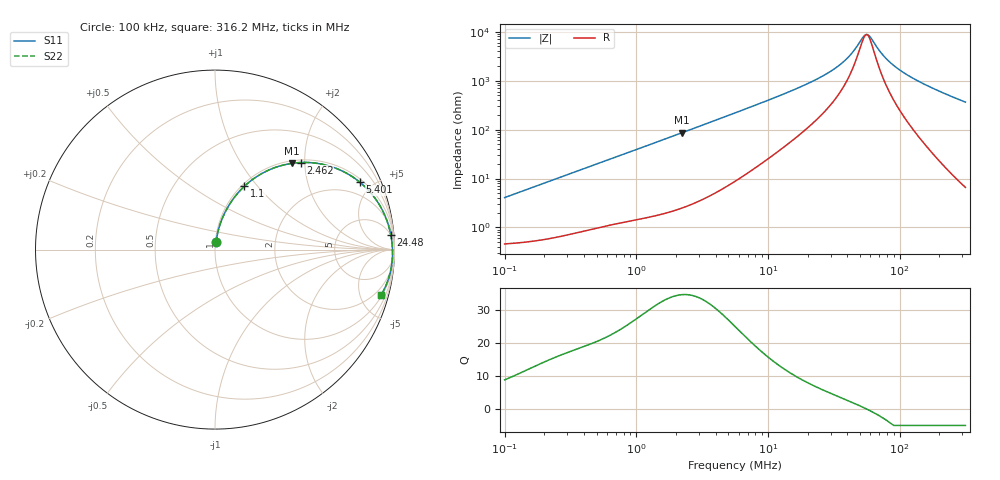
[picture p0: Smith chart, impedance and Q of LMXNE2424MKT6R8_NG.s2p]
! LMXNE2424MKT6R8_NG  S-PARAMETER MODEL  ( General Type )
! Model Generated by TAIYO YUDEN Corporation (https://www.yuden.co.jp/en/)
! Version 1.0
! TAIYO YUDEN Control No. 191023NI43SB-FBB
! Copyright(c) 2019 TAIYO YUDEN CO.,LTD. All Rights Reserved.
! Product Description (link to TY-COMPAS)
! https://ds.yuden.co.jp/TYCOMPAS/or/detail?pn=LMXNE2424MKT6R8MNG&u=M
! Products Name : Inductors
! Characteristics :
!  Inductance : 6.8 uH , SRF(min) : 34 MHz , DC Resistance(max) : 0.504 Ohm
!  Rated Current : Saturation :950 mA , Temp Rise : 550 mA (40 degC)
!  Case Size : 2.4 x 2.4 / 0.095 x 0.095 [mm/inch] , Thickness : 1.2 / 0.047 [mm/inch]
!  (Conditions: Temperature = 25 degC , DC Bias Current/Voltage = 0A / 0V)
! External Node Assignments :
!  1  o---GGG---o  2
! GND o---------o GND
! Frequency Range : 0.1MHz  -  316.199832MHz  [ 402 STEP ]
# MHz S RI R 50
! Freq[MHz].  S11 Real  S11 Imag  S21 Real  S21 Imag  S12 Real  S12 Imag  S22 Real  S22 Imag
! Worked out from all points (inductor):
!   401 points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, 100 kHz to 316.2 MHz, reference 50 ohm
!   read as one part in series: L = 6.44 uH near 104.1 kHz
!   highest Q = 34.6 at 2.226 MHz (marker M1), where L = 6.17 uH
!   self-resonance near 55.91 MHz
!   S11 on the Smith chart (normalised r, x): 100 kHz: 1.01, +0.08; 1.1 MHz: 1.03, +0.86; 2.462 MHz: 1.06, +1.91; 5.401 MHz: 1.16, +4.20; 24.48 MHz: 5, +22; 316.2 MHz: 1.13, -7.28
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0.1  0.0062 0.0401  0.9938 -0.0401  0.9938 -0.0401  0.0062 0.0401
0.385695  0.0307 0.1477  0.9693 -0.1477  0.9693 -0.1477  0.0307 0.1477
1.09961  0.1638 0.3529  0.8362 -0.3529  0.8362 -0.3529  0.1638 0.3529
1.487603  0.257 0.4216  0.743 -0.4216  0.743 -0.4216  0.257 0.4216
2.225795  0.4289 0.4807  0.5711 -0.4807  0.5711 -0.4807  0.4289 0.4807
2.461698  0.4773 0.4853  0.5227 -0.4853  0.5227 -0.4853  0.4773 0.4853
3.467234  0.6399 0.4648  0.3601 -0.4648  0.3601 -0.4648  0.6399 0.4648
5.401085  0.8064 0.3761  0.1936 -0.3761  0.1936 -0.3761  0.8064 0.3761
5.623165  0.818 0.3663  0.182 -0.3663  0.182 -0.3663  0.818 0.3663
9.885033  0.9261 0.232  0.0739 -0.232  0.0739 -0.232  0.9261 0.232
21.68824  0.976 0.0989  0.024 -0.0989  0.024 -0.0989  0.976 0.0989
24.47506  0.9791 0.0839  0.0209 -0.0839  0.0209 -0.0839  0.9791 0.0839
38.12604  0.9862 0.0364  0.0138 -0.0364  0.0138 -0.0364  0.9862 0.0364
43.90066  0.9875 0.0229  0.0125 -0.0229  0.0125 -0.0229  0.9875 0.0229
52.6284  0.9885 0.00588  0.0115 -0.00588  0.0115 -0.00588  0.9885 0.00588
55.90748  0.9888 0.000242  0.0112 -0.000242  0.0112 -0.000242  0.9888 0.000242
59.39086  0.9889 -0.00542  0.0111 0.00542  0.0111 0.00542  0.9889 -0.00542
72.64716  0.9891 -0.0247  0.0109 0.0247  0.0109 0.0247  0.9891 -0.0247
83.65039  0.9887 -0.0389  0.0113 0.0389  0.0113 0.0389  0.9887 -0.0389
104.4039  0.9871 -0.0632  0.0129 0.0632  0.0129 0.0632  0.9871 -0.0632
138.4253  0.9824 -0.099  0.0176 0.099  0.0176 0.099  0.9824 -0.099
316.1998  0.926 -0.2529  0.074 0.2529  0.074 0.2529  0.926 -0.2529
